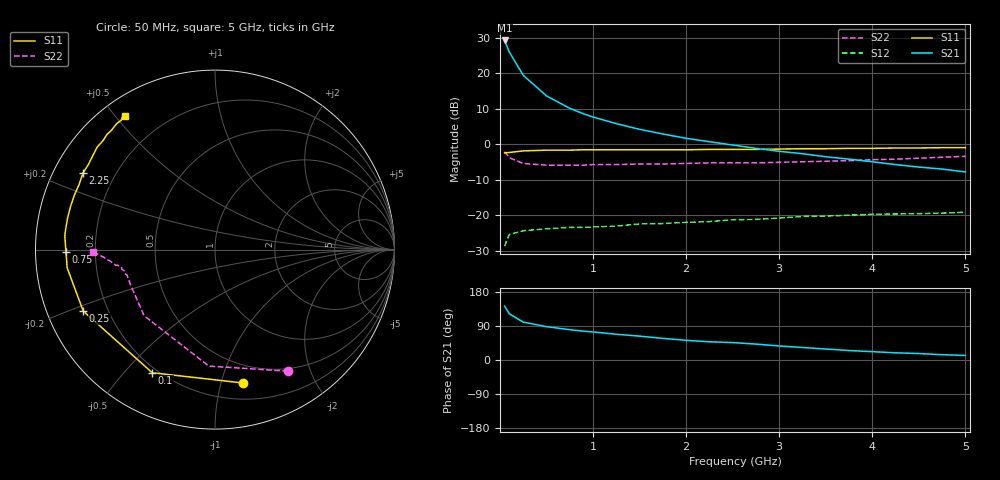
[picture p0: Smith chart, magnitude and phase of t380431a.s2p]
!AT-38043
!S-PARAMETERS at Vce=1.2V Ic=50mA. LAST UPDATED 01-06-98
# ghz s ma r 50
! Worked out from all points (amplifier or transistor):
!   23 points, 50 MHz to 5 GHz, reference 50 ohm
!   highest |S21| = 29.3 dB at 50 MHz (marker M1)
!   |S21| within 3 dB of that: start of sweep to 96.43 MHz
!   unconditionally stable (mu >= 1): 1.623 GHz to end of sweep
!   at 500 MHz: K = 0.41, MSG = 18.7 dB, |S12| = -23.7 dB
!   at 2.25 GHz: K = 1.22, MAG = 8.4 dB, |S12| = -21.7 dB
!   at 5 GHz: K = 1.32, MAG = 2.3 dB, |S12| = -19.1 dB
!   S11 on the Smith chart (normalised r, x): 50 MHz: 0.33, -1.18; 100 MHz: 0.18, -0.60; 250 MHz: 0.11, -0.22; 750 MHz: 0.09, -0.01; 2.25 GHz: 0.09, +0.27; 5 GHz: 0.07, +0.53
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0.05  0.76 -78.0  29.01 142.0  0.037 51.0  0.79 -59.0
0.1  0.77 -117.0  20 122.0  0.054 35.0  0.65 -93.0
0.25  0.81 -155.0  9.39 100.0  0.061 20.0  0.54 -137.0
0.5  0.83 -173.0  4.81 88.0  0.065 18.0  0.51 -156.0
0.75  0.83 -179.0  3.22 80.0  0.068 19.0  0.51 -162.0
0.9  0.84 175.0  2.69 76.0  0.068 20.0  0.51 -164.0
1  0.84 173.0  2.43 74.0  0.069 22.0  0.52 -165.0
1.25  0.84 168.0  1.96 68.0  0.071 24.0  0.52 -167.0
1.5  0.84 163.0  1.63 63.0  0.076 25.0  0.53 -168.0
1.75  0.84 159.0  1.4 57.0  0.077 27.0  0.53 -169.0
2  0.84 154.0  1.22 52.0  0.08 31.0  0.54 -170.0
2.25  0.85 150.0  1.09 48.0  0.082 33.0  0.55 -171.0
2.5  0.85 149.0  0.98 46.0  0.087 36.0  0.55 -171.0
2.75  0.85 146.0  0.88 42.0  0.088 37.0  0.55 -171.0
3  0.86 142.0  0.8 37.0  0.092 39.0  0.56 -171.0
3.25  0.87 139.0  0.74 33.0  0.097 40.0  0.57 -172.0
3.5  0.87 136.0  0.67 29.0  0.098 40.0  0.58 -173.0
3.75  0.88 133.0  0.62 25.0  0.101 41.0  0.59 -174.0
4  0.88 131.0  0.57 22.0  0.104 41.0  0.61 -175.0
4.25  0.89 128.0  0.52 19.0  0.105 40.0  0.62 -176.0
4.5  0.89 126.0  0.48 17.0  0.106 40.0  0.64 -177.0
5  0.9 124.0  0.41 12.0  0.111 40.0  0.68 -179.0
